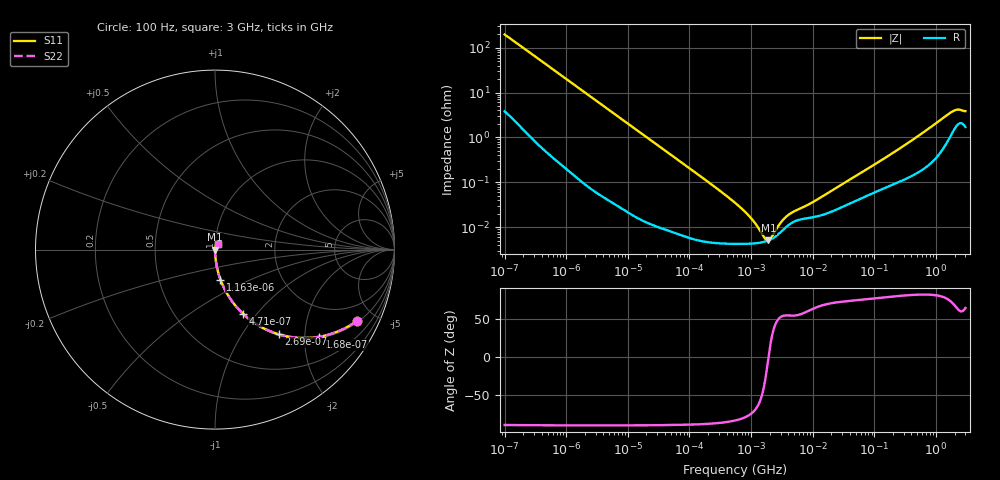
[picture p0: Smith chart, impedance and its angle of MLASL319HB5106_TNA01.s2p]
! MLASL319HB5106_TNA01  S-PARAMETER MODEL  ( Standard Model )
! Model Generated by TAIYO YUDEN Corporation (http://www.ty-top.com)
! Version 1.0
! TAIYO YUDEN Control No. 220601
! Copyright(c) 2009 TAIYO YUDEN CO.,LTD. All Rights Reserved.
! Product Description (link to TY-COMPAS)
! https://ds.yuden.co.jp/TYCOMPAS/or/detail?pn=MLASL319HB5106KTNA01&u=M
! Products Name : Multilayer Ceramic Capacitors
! Characteristics :
!  Capacitance : 10 [uF] , Rated Voltage : 10 [V] , TCC : X5R
!  Case Size : 3.2 x 1.6 / 0.126 x 0.063 [mm/inch] , Thickness : 0.85 / 0.033 [mm/inch]
!  (Conditions: Temperature = 25 [degC] , DC Bias Voltage = 0 [V])
! External Node Assignments :
!  1  o---| |---o  2
! GND o---------o GND
! Frequency Range : 100Hz  -  3GHz  [ 401 STEP ]
# MHZ S RI R 50
! Freq[MHz].  S11 Real  S11 Imag  S21 Real  S21 Imag  S12 Real  S12 Imag  S22 Real  S22 Imag
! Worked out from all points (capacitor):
!   401 points, 100 Hz to 3 GHz, reference 50 ohm
!   read as one part in series: C = 8.07 uF near 109 Hz
!   lowest |Z| = 5.06 mohm at 1.908 MHz (marker M1)
!   series resonance near 1.919 MHz, so ESL is about 850 pH
!   S11 on the Smith chart (normalised r, x): 100 Hz: 1.08, -3.93; 168 Hz: 1.04, -2.36; 269 Hz: 1.02, -1.48; 471 Hz: 1.01, -0.85; 1.163 kHz: 1.00, -0.34; 3 GHz: 1.03, +0.07
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0.0001  0.7898 -0.3979  0.2102 0.3979  0.2102 0.3979  0.7898 -0.3979
0.000168  0.5811 -0.4853  0.4189 0.4853  0.4189 0.4853  0.5811 -0.4853
0.000269  0.3548 -0.4718  0.6452 0.4718  0.6452 0.4718  0.3548 -0.4718
0.000471  0.1549 -0.3562  0.8451 0.3562  0.8451 0.3562  0.1549 -0.3562
0.000724  0.0731 -0.2552  0.9269 0.2552  0.9269 0.2552  0.0731 -0.2552
0.001163  0.0304 -0.1669  0.9696 0.1669  0.9696 0.1669  0.0304 -0.1669
0.001788  0.0134 -0.1107  0.9866 0.1107  0.9866 0.1107  0.0134 -0.1107
0.005476  0.00171 -0.0368  0.9983 0.0368  0.9983 0.0368  0.00171 -0.0368
0.031977  0.000139 -0.00637  0.9999 0.00637  0.9999 0.00637  0.000139 -0.00637
0.221826  4.62e-05 -0.000918  1 0.000918  1 0.000918  4.62e-05 -0.000918
0.547723  4.25e-05 -0.000348  1 0.000348  1 0.000348  4.25e-05 -0.000348
0.842342  4.26e-05 -0.0002  1 0.0002  1 0.0002  4.26e-05 -0.0002
1.295438  4.44e-05 -8.82e-05  1 8.82e-05  1 8.82e-05  4.44e-05 -8.82e-05
1.908323  5.06e-05 -1.17e-06  0.9999 1.17e-06  0.9999 1.17e-06  5.06e-05 -1.17e-06
2.579298  6.44e-05 6.54e-05  0.9999 -6.54e-05  0.9999 -6.54e-05  6.44e-05 6.54e-05
3.639519  9.82e-05 0.000135  0.9999 -0.000135  0.9999 -0.000135  9.82e-05 0.000135
4.323298  0.000119 0.000162  0.9999 -0.000162  0.9999 -0.000162  0.000119 0.000162
9.794414  0.000165 0.000314  0.9998 -0.000314  0.9998 -0.000314  0.000165 0.000314
175.1444  0.000838 0.00393  0.9992 -0.00393  0.9992 -0.00393  0.000838 0.00393
1789.813  0.0128 0.0341  0.9872 -0.0341  0.9872 -0.0341  0.0128 0.0341
2219.584  0.0199 0.0357  0.9801 -0.0357  0.9801 -0.0357  0.0199 0.0357
3000  0.0179 0.0333  0.9821 -0.0333  0.9821 -0.0333  0.0179 0.0333
